(* Logix 5000 AddOnInstructionDefinition export Banner_TL50Select_Param_v4; software revision 33.00 *)

TYPE Banner_IOL_Port_v4 :   // UDT that has all of the data items necessary to communicate with a specific Port on a IO-Link Master
STRUCT
   Port_Controlled : INT;   // Each bit represents a port on an IO-Link Master. Set to 1 to tell AOI to control that port.
   Port_Activate : INT;   // Each bit represents a port on an IO-Link Master. When ON that port will process any commands in queue.
   Port_Read : INT;   // Each bit represents a port on an IO-Link Master. Used to determine when device AOI has requested a Read command.
   Port_Write : INT;   // Each bit represents a port on an IO-Link Master. Used to determine when device AOI has requested a Write command.
   Port_RW_Complete : INT;   // Each bit represents a port on an IO-Link Master. Tells device AOI that Read or Write request has been completed.
   Port_Device_Read : INT;
   Data_Transfer : SINT[190];   // Array to transfer data from IO-Master to device AOIs.
END_STRUCT
END_TYPE

TYPE Banner_TL50Select_Basic_SP_v4 :   // Basic parameters for a TL50 Pro Select segment.
STRUCT
   Basic_Color : SINT;   // 0 = Green, 1 = Red, 2 = Orange, 3 = Amber, 4 = Yellow, 5 = Lime Green, 6 = Spring Green, 7 = Cyan, 8 = Sky Blue, 9 = Blue, 10 = Violet, 11 = Magenta, 12 = Rose, 13 = White, 14 = Custom, 15 = Custom 2
   Basic_Speed : SINT;   // 0 = Medium, 1 = Fast, 2 = Slow, 3 = Custom
   Animation : SINT;   // 0 = Off, 1 = Steady, 2 = Flash, 3 = Two Color, 4 = Half/Half, 5 = Half/Half Rotate, 6 = Chase, 7 = Intesnity Sweep
   Animation_Color_1 : INT;   // 0 = Green, 1 = Red, 2 = Orange, 3 = Amber, 4 = Yellow, 5 = Lime Green, 6 = Spring Green, 7 = Cyan, 8 = Sky Blue, 9 = Blue, 10 = Violet, 11 = Magenta, 12 = Rose, 13 = White, 14 = Custom, 15 = Custom 2
   Animation_Color_1_Intensity : SINT;   // 0 = High, 1 = Low, 2 = Medium, 3 = Off, 4 = Custom
   Animation_Speed : SINT;   // 0 = Medium, 1 = Fasr, 2 = Slow, 3 = Custom
   Animation_Pattern : SINT;   // 0 = Normal, 1 = Strobe, 2 = Three Pulse, 3 = SOS, 4 = Random
   Animation_Color_2 : INT;   // 0 = Green, 1 = Red, 2 = Orange, 3 = Amber, 4 = Yellow, 5 = Lime Green, 6 = Spring Green, 7 = Cyan, 8 = Sky Blue, 9 = Blue, 10 = Violet, 11 = Magenta, 12 = Rose, 13 = White, 14 = Custom, 15 = Custom 2
   Animation_Color_2_Intensity : SINT;   // 0 = High, 1 = Low, 2 = Medium, 3 = Off, 4 = Custom
END_STRUCT
END_TYPE

TYPE Banner_TL50Select_RD_v4 :   // UDT that stores the Read Data for a TL50 Pro Select.
STRUCT
   Master_Cycle_Time : INT;
   Min_Cycle_Time : INT;
   M_Sequence_Capability : INT;
   IO_Link_Version_ID : INT;
   Process_Data_Input_Length : INT;
   Process_Data_Output_Length : INT;
   Combined_Vendor_ID : DINT;   // IO-Link Vendor ID
   Vendor_ID1 : INT;
   Vendor_ID2 : INT;
   Combined_Device_ID : DINT;   // IO-Link Device ID
   Device_ID1 : INT;
   Device_ID2 : INT;
   Device_ID3 : INT;
   Serial_Number : STRING;
END_STRUCT
END_TYPE

TYPE Banner_TL50Select_v4 :   // All of the parameters for a TL50 Pro Select.
STRUCT
   Initial_Global_Read : BOOL;   // Determines if all of the IO-Link data has been read into the PLC yet
   Command : INT;   // Value placed in here will activate a read or write to a specifc IO-Link Index
   Read : Banner_TL50Select_RD_v4;   // Read Only Data
   Write : Banner_TL50Select_WD_v4;   // Write Data
   Archive_Data : Banner_TL50Select_WD_v4;   // Archive of the Write Data
   Reset : BOOL;   // Resets AOI. This will force a complete parameter read of the sensor.
END_STRUCT
END_TYPE

TYPE Banner_TL50Select_WD_v4 :   // UDT that stores the Write Data for a TL50 Pro Select.
STRUCT
   System_Command : INT;   // See IODD file for list of commands that can be activated via the System Command interface
   Parameter_Access_Lock : SINT;   // Write access to all parameters is prohibited while value is 1. Only this parameter can be adjusted when value is 1.
   Data_Storage_Lock : SINT;   // Automatic data storage is disabled when this value is equal to 1. Read access is not affected.
   Local_Parameterization_Lock : SINT;   // Parameterization via local control elements on device is disabled.
   Local_User_Interface_Lock : SINT;   // Operation of local user interface is disabled.
   Operating_Mode_Selection : SINT;   // 0 = Basic Mode, 1 = Advanced Mode, 2= Run Mode, 3 = Level Mode
   Segment_Basic : Banner_TL50Select_Basic_SP_v4[5];
   Restrict_to_Gamut : SINT;   // 0 = Off, 1 = On
   Number_of_Segments_for_Scroll_and_Bounce : INT;   // 0 to 10
   Custom_Flash_Rate : INT;   // .5 to 20 Hz (range 5 to 200)
   Custom_Intensity : INT;   // 0 to 100%
   Custom_1_Red : INT;   // 0 to 255. Value of the Red portion of the RGB color value for Custom 1
   Custom_1_Green : INT;   // 0 to 255. Value of the Green portion of the RGB color value for Custom 1.
   Custom_1_Blue : INT;   // 0 to 255. Value of the Blue portion of the RGB color value for Custom 1.
   Custom_2_Red : INT;   // 0 to 255. Value of the Red portion of the RGB color value for Custom 2.
   Custom_2_Green : INT;   // 0 to 255. Value of the Green portion of the RGB color value for Custom 2.
   Custom_2_Blue : INT;   // 0 to 255. Value of the Blue portion of the RGB color value for Custom 2.
   LM_Full_Scale_Value : DINT;
   LM_Base_Color : INT;   // 0 = Green, 1 = Red, 2 = Orange, 3 = Amber, 4 = Yellow, 5 = Lime Green, 6 = Spring Green, 7 = Cyan, 8 = Sky Blue, 9 = Blue, 10 = Violet, 11 = Magenta, 12 = Rose, 13 = White, 14 = Custom, 15 = Custom 2
   LM_Base_Intensity : SINT;   // 0 = High, 1 = Low, 2 = Medium, 3 = Off, 4 = Custom
   LM_Base_State : SINT;   // 0 = Steady, 1 = Flashing
   LM_Threshold_Type : SINT;   // 0 = None, 1 = Low, 2 = High, 3 = High and Low
   LM_Low_Threshold_Value : DINT;
   LM_Low_Threshold_Color : INT;   // 0 = Green, 1 = Red, 2 = Orange, 3 = Amber, 4 = Yellow, 5 = Lime Green, 6 = Spring Green, 7 = Cyan, 8 = Sky Blue, 9 = Blue, 10 = Violet, 11 = Magenta, 12 = Rose, 13 = White, 14 = Custom, 15 = Custom 2
   LM_Low_Threshold_Intensity : SINT;   // 0 = High, 1 = Low, 2 = Medium, 3 = Off, 4 = Custom
   LM_Low_Threshold_State : SINT;   // 0 = Steady, 1 = Flashing
   LM_High_Threshold_Value : DINT;
   LM_High_Threshold_Color : INT;   // 0 = Green, 1 = Red, 2 = Orange, 3 = Amber, 4 = Yellow, 5 = Lime Green, 6 = Spring Green, 7 = Cyan, 8 = Sky Blue, 9 = Blue, 10 = Violet, 11 = Magenta, 12 = Rose, 13 = White, 14 = Custom, 15 = Custom 2
   LM_High_Threshold_Intensity : SINT;   // 0 = High, 1 = Low, 2 = Medium, 3 = Off, 4 = Custom
   LM_High_Threshold_State : SINT;   // 0 = Steady, 1 = Flashing
   LM_Flash_Rate : SINT;   // 0 = Medium, 1 = Fast, 2 = Slow, 3 = Custom
   LM_Dominance : SINT;   // 0 = Dominant, 1 = Non-Dominant
   LM_Subsegment_Style : SINT;   // 0 = Steady, 1 = Flashing, 2 = Analog
   LM_Background_Color : SINT;   // 0 = Green, 1 = Red, 2 = Orange, 3 = Amber, 4 = Yellow, 5 = Lime Green, 6 = Spring Green, 7 = Cyan, 8 = Sky Blue, 9 = Blue, 10 = Violet, 11 = Magenta, 12 = Rose, 13 = White, 14 = Custom, 15 = Custom 2
   LM_Background_Intensity : SINT;   // 0 = High, 1 = Low, 2 = Medium, 3 = Off, 4 = Custom
   LM_Orientation : SINT;   // 0 = Steady, 1 = Flashing
END_STRUCT
END_TYPE

ADD_ON_INSTRUCTION Banner_TL50Select_Param_v4   (* revision 4.1, vendor Banner Engineering *)
// AOI to read and write parameter data to an IO-Link TL50 Pro Select.
VAR_IN_OUT
   TL50_Pro : Banner_TL50Select_v4; {required}
   Port_Data : Banner_IOL_Port_v4; {required}
END_VAR
VAR_INPUT
   Port : INT; {required}   // Port Number that device is plugged into.
END_VAR
VAR
   Local_Control : DINT; {access None}
   Global_Read_Command_Value : INT; {access None}
   Global_Write_Command_Value : INT; {access None}
   Command_Being_Processed : BOOL; {access None}
   Update_Archive : BOOL; {access None}
   Index_Write_Inprocess : DINT; {access None}
   Index_Write_Control : DINT; {access None}
   Inprocess_Index : DINT; {access None}
   Index_R_Segment : DINT; {access None}
   BS_Index : DINT; {access None}
   Index_W_Segment : DINT; {access None}
   SB_W_Index : DINT; {access None}
   Index_Segment_Read : DINT; {access None}
END_VAR

ROUTINE Logic   (* ladder *)
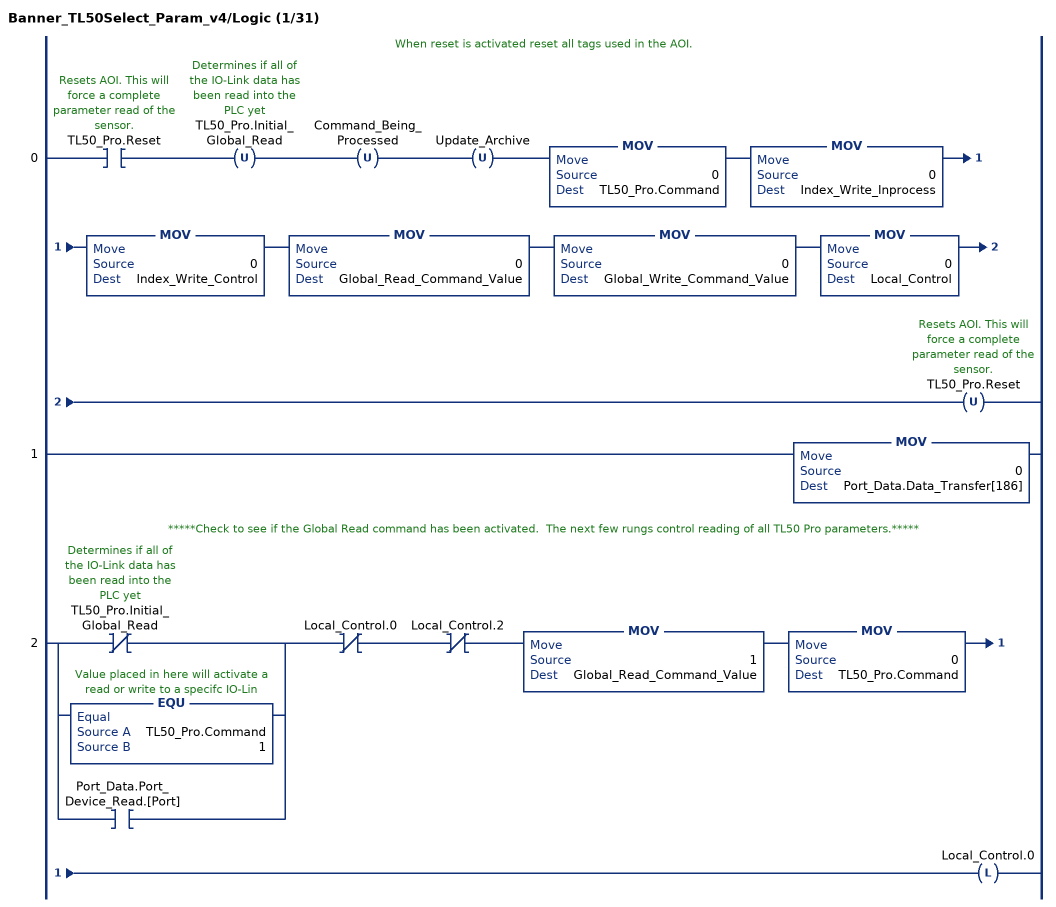
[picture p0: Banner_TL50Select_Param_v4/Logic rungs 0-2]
   // When reset is activated reset all tags used in the AOI.
   0: XIC(TL50_Pro.Reset)OTU(TL50_Pro.Initial_Global_Read)OTU(Command_Being_Processed)OTU(Update_Archive)MOV(0,TL50_Pro.Command)MOV(0,Index_Write_Inprocess)MOV(0,Index_Write_Control)MOV(0,Global_Read_Command_Value)MOV(0,Global_Write_Command_Value)MOV(0,Local_Control)OTU(TL50_Pro.Reset);
   1: MOV(0,Port_Data.Data_Transfer[186]);
   // *****Check to see if the Global Read command has been activated.  The next few rungs control reading of all TL50 Pro parameters.*****
   2: [XIO(TL50_Pro.Initial_Global_Read) ,EQU(TL50_Pro.Command,1) ,XIC(Port_Data.Port_Device_Read.[Port]) ]XIO(Local_Control.0)XIO(Local_Control.2)MOV(1,Global_Read_Command_Value)MOV(0,TL50_Pro.Command)OTL(Local_Control.0);
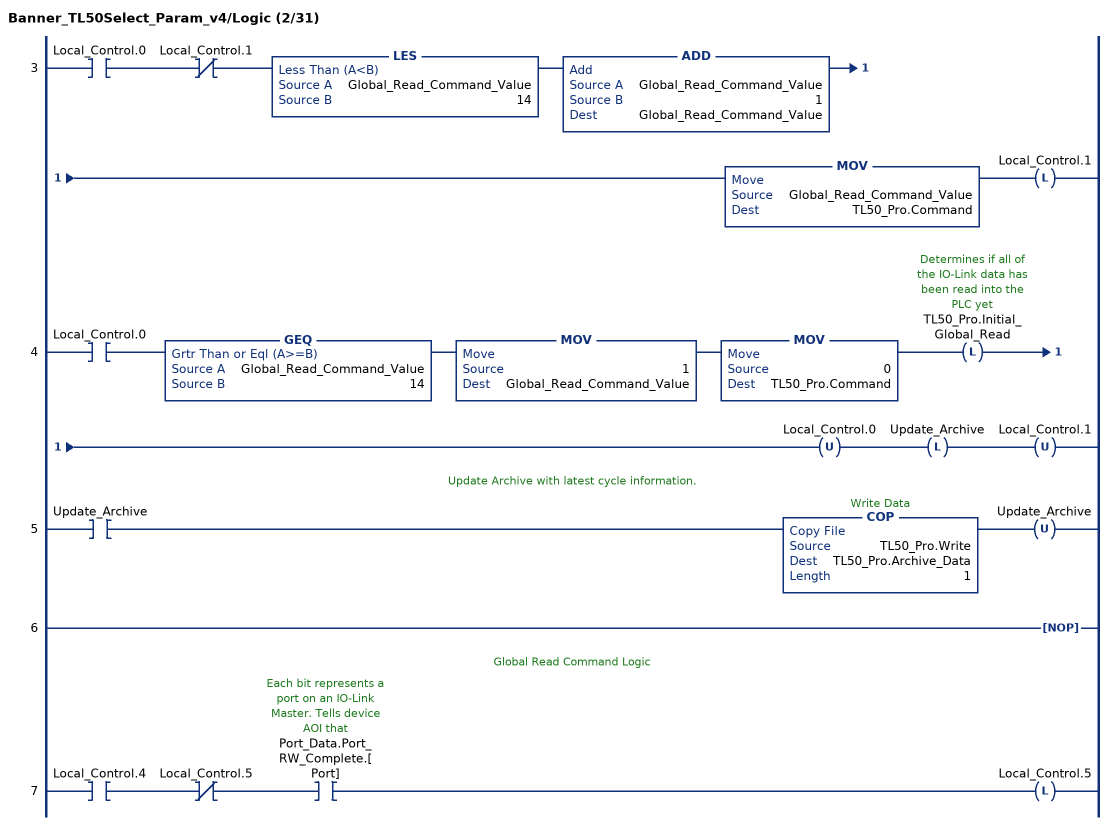
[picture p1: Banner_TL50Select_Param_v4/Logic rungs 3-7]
   3: XIC(Local_Control.0)XIO(Local_Control.1)LES(Global_Read_Command_Value,14)ADD(Global_Read_Command_Value,1,Global_Read_Command_Value)MOV(Global_Read_Command_Value,TL50_Pro.Command)OTL(Local_Control.1);
   4: XIC(Local_Control.0)GEQ(Global_Read_Command_Value,14)MOV(1,Global_Read_Command_Value)MOV(0,TL50_Pro.Command)OTL(TL50_Pro.Initial_Global_Read)OTU(Local_Control.0)OTL(Update_Archive)OTU(Local_Control.1);
   // Update Archive with latest cycle information.
   5: XIC(Update_Archive)COP(TL50_Pro.Write,TL50_Pro.Archive_Data,1)OTU(Update_Archive);
   6: NOP();
   // Global Read Command Logic
   7: XIC(Local_Control.4)XIO(Local_Control.5)XIC(Port_Data.Port_RW_Complete.[Port])OTL(Local_Control.5);
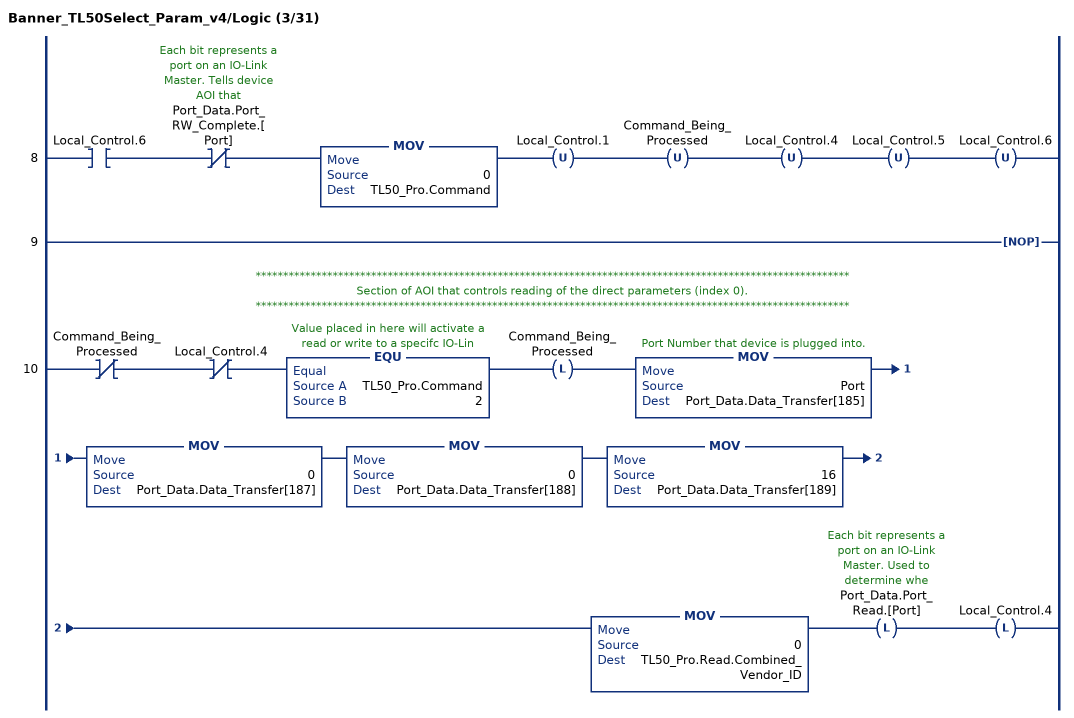
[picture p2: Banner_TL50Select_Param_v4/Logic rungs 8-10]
   8: XIC(Local_Control.6)XIO(Port_Data.Port_RW_Complete.[Port])MOV(0,TL50_Pro.Command)OTU(Local_Control.1)OTU(Command_Being_Processed)OTU(Local_Control.4)OTU(Local_Control.5)OTU(Local_Control.6);
   9: NOP();
   // ************************************************************************************************************
   // Section of AOI that controls reading of the direct parameters (index 0).
   // ************************************************************************************************************
   10: XIO(Command_Being_Processed)XIO(Local_Control.4)EQU(TL50_Pro.Command,2)OTL(Command_Being_Processed)MOV(Port,Port_Data.Data_Transfer[185])MOV(0,Port_Data.Data_Transfer[187])MOV(0,Port_Data.Data_Transfer[188])MOV(16,Port_Data.Data_Transfer[189])MOV(0,TL50_Pro.Read.Combined_Vendor_ID)OTL(Port_Data.Port_Read.[Port])OTL(Local_Control.4);
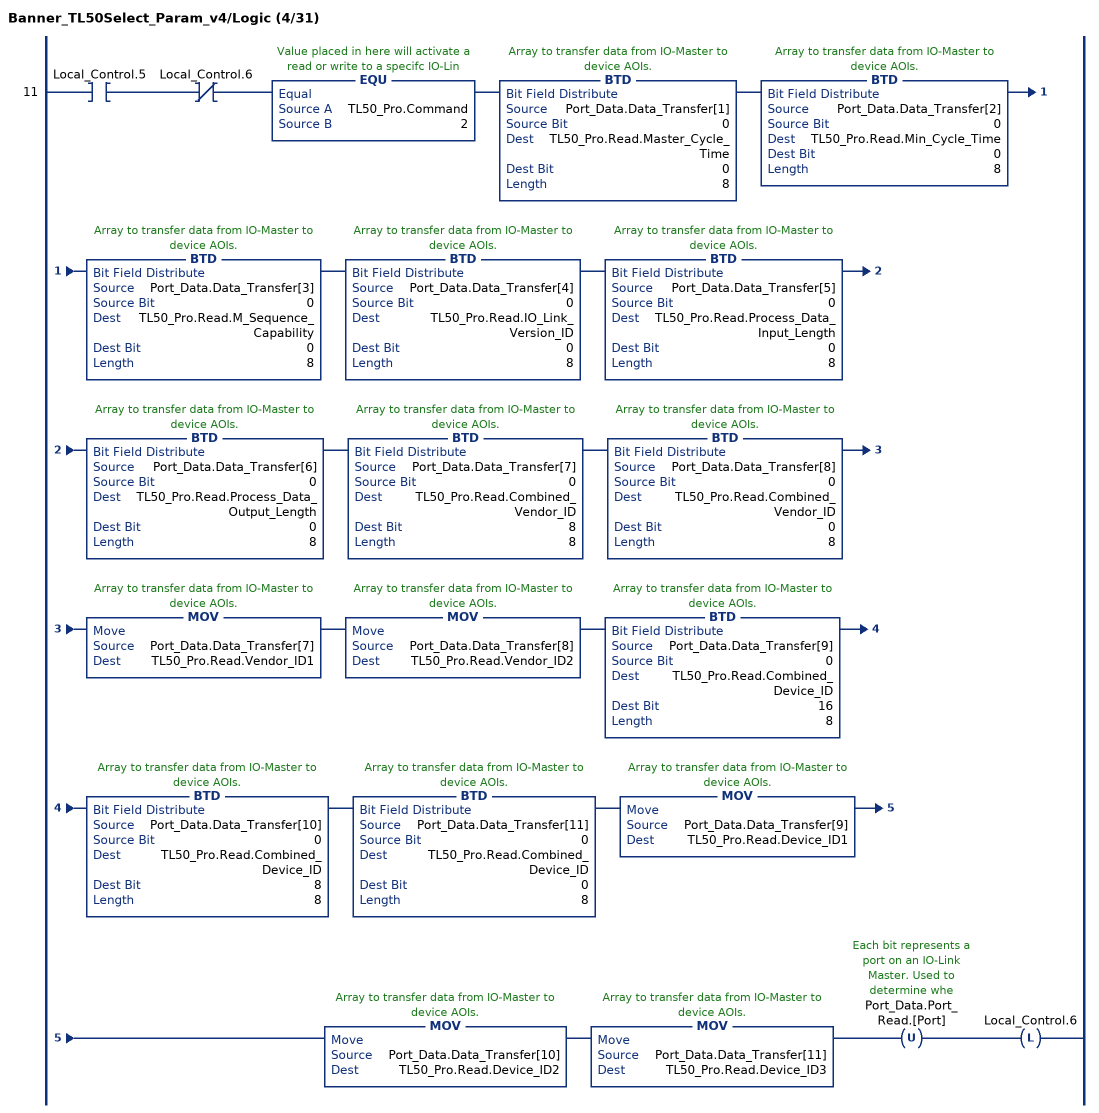
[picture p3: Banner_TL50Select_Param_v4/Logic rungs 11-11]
   11: XIC(Local_Control.5)XIO(Local_Control.6)EQU(TL50_Pro.Command,2)BTD(Port_Data.Data_Transfer[1],0,TL50_Pro.Read.Master_Cycle_Time,0,8)BTD(Port_Data.Data_Transfer[2],0,TL50_Pro.Read.Min_Cycle_Time,0,8)BTD(Port_Data.Data_Transfer[3],0,TL50_Pro.Read.M_Sequence_Capability,0,8)BTD(Port_Data.Data_Transfer[4],0,TL50_Pro.Read.IO_Link_Version_ID,0,8)BTD(Port_Data.Data_Transfer[5],0,TL50_Pro.Read.Process_Data_Input_Length,0,8)BTD(Port_Data.Data_Transfer[6],0,TL50_Pro.Read.Process_Data_Output_Length,0,8)BTD(Port_Data.Data_Transfer[7],0,TL50_Pro.Read.Combined_Vendor_ID,8,8)BTD(Port_Data.Data_Transfer[8],0,TL50_Pro.Read.Combined_Vendor_ID,0,8)MOV(Port_Data.Data_Transfer[7],TL50_Pro.Read.Vendor_ID1)MOV(Port_Data.Data_Transfer[8],TL50_Pro.Read.Vendor_ID2)BTD(Port_Data.Data_Transfer[9],0,TL50_Pro.Read.Combined_Device_ID,16,8)BTD(Port_Data.Data_Transfer[10],0,TL50_Pro.Read.Combined_Device_ID,8,8)BTD(Port_Data.Data_Transfer[11],0,TL50_Pro.Read.Combined_Device_ID,0,8)MOV(Port_Data.Data_Transfer[9],TL50_Pro.Read.Device_ID1)MOV(Port_Data.Data_Transfer[10],TL50_Pro.Read.Device_ID2)MOV(Port_Data.Data_Transfer[11],TL50_Pro.Read.Device_ID3)OTU(Port_Data.Port_Read.[Port])OTL(Local_Control.6);
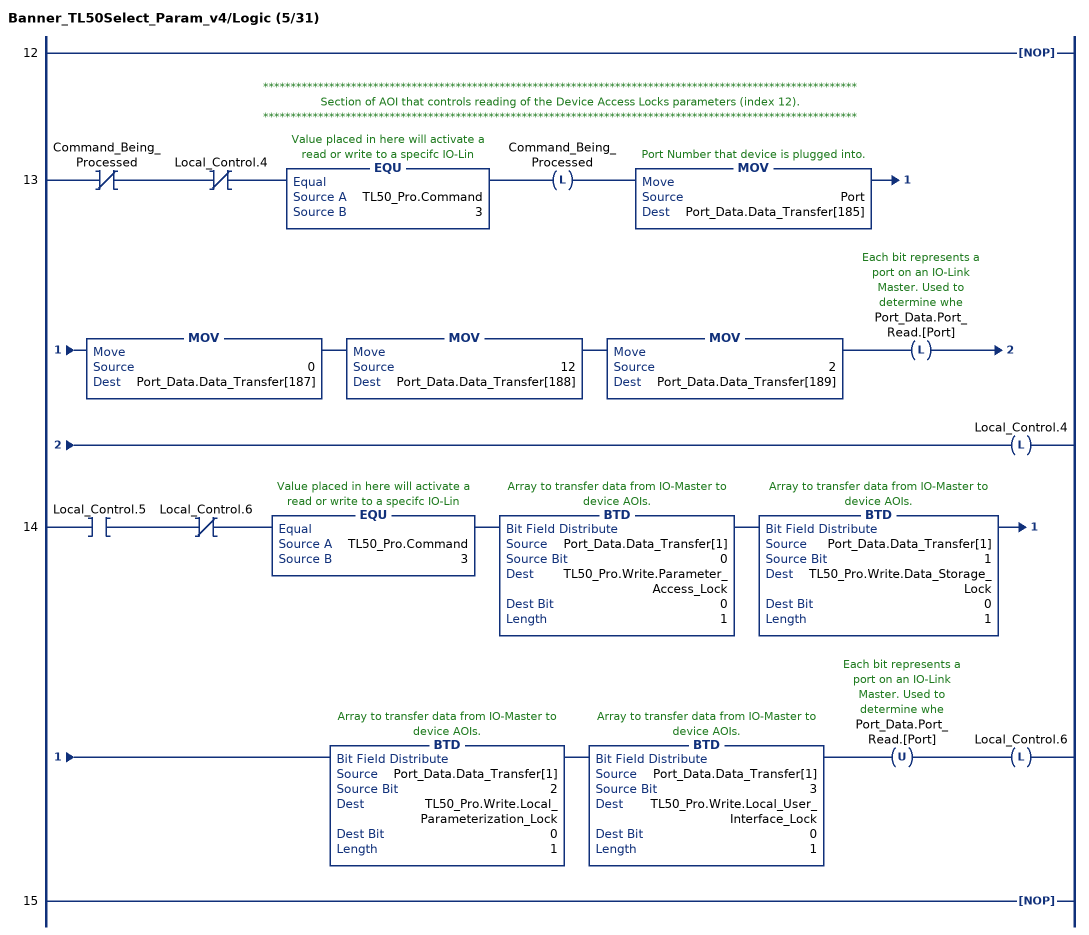
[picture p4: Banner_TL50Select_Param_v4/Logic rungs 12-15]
   12: NOP();
   // ************************************************************************************************************
   // Section of AOI that controls reading of the Device Access Locks parameters (index 12).
   // ************************************************************************************************************
   13: XIO(Command_Being_Processed)XIO(Local_Control.4)EQU(TL50_Pro.Command,3)OTL(Command_Being_Processed)MOV(Port,Port_Data.Data_Transfer[185])MOV(0,Port_Data.Data_Transfer[187])MOV(12,Port_Data.Data_Transfer[188])MOV(2,Port_Data.Data_Transfer[189])OTL(Port_Data.Port_Read.[Port])OTL(Local_Control.4);
   14: XIC(Local_Control.5)XIO(Local_Control.6)EQU(TL50_Pro.Command,3)BTD(Port_Data.Data_Transfer[1],0,TL50_Pro.Write.Parameter_Access_Lock,0,1)BTD(Port_Data.Data_Transfer[1],1,TL50_Pro.Write.Data_Storage_Lock,0,1)BTD(Port_Data.Data_Transfer[1],2,TL50_Pro.Write.Local_Parameterization_Lock,0,1)BTD(Port_Data.Data_Transfer[1],3,TL50_Pro.Write.Local_User_Interface_Lock,0,1)OTU(Port_Data.Port_Read.[Port])OTL(Local_Control.6);
   15: NOP();
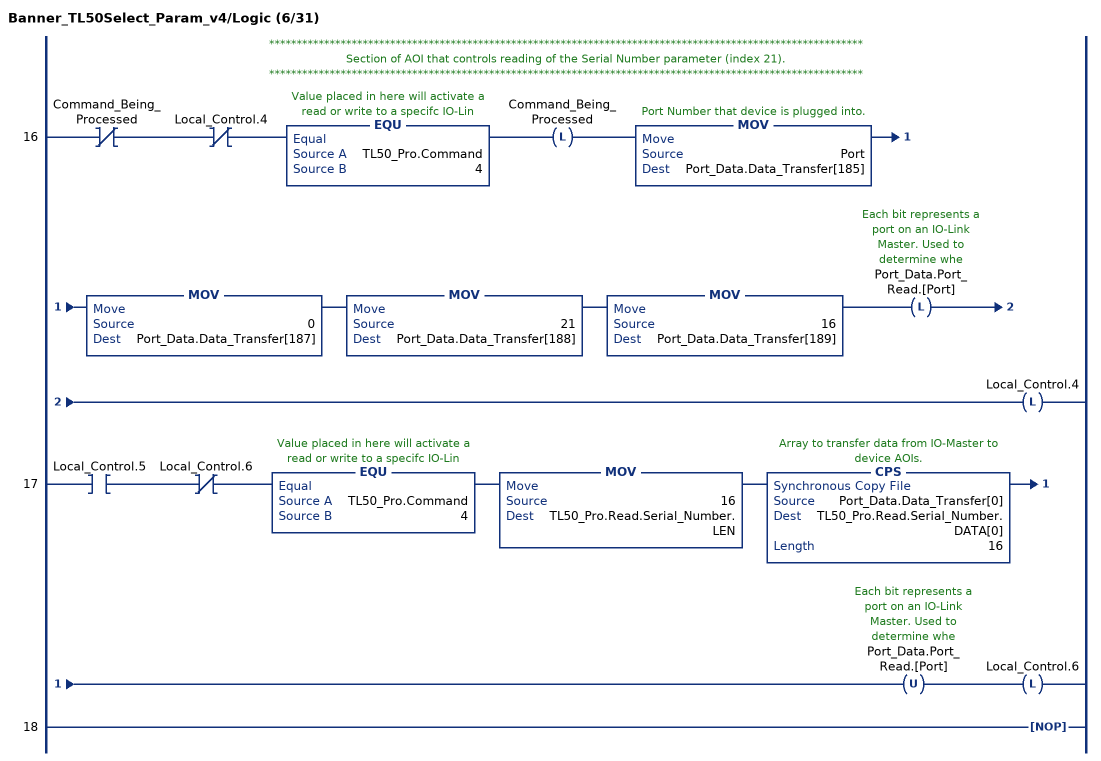
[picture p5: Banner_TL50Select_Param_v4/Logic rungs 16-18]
   // ************************************************************************************************************
   // Section of AOI that controls reading of the Serial Number parameter (index 21).
   // ************************************************************************************************************
   16: XIO(Command_Being_Processed)XIO(Local_Control.4)EQU(TL50_Pro.Command,4)OTL(Command_Being_Processed)MOV(Port,Port_Data.Data_Transfer[185])MOV(0,Port_Data.Data_Transfer[187])MOV(21,Port_Data.Data_Transfer[188])MOV(16,Port_Data.Data_Transfer[189])OTL(Port_Data.Port_Read.[Port])OTL(Local_Control.4);
   17: XIC(Local_Control.5)XIO(Local_Control.6)EQU(TL50_Pro.Command,4)MOV(16,TL50_Pro.Read.Serial_Number.LEN)CPS(Port_Data.Data_Transfer[0],TL50_Pro.Read.Serial_Number.DATA[0],16)OTU(Port_Data.Port_Read.[Port])OTL(Local_Control.6);
   18: NOP();
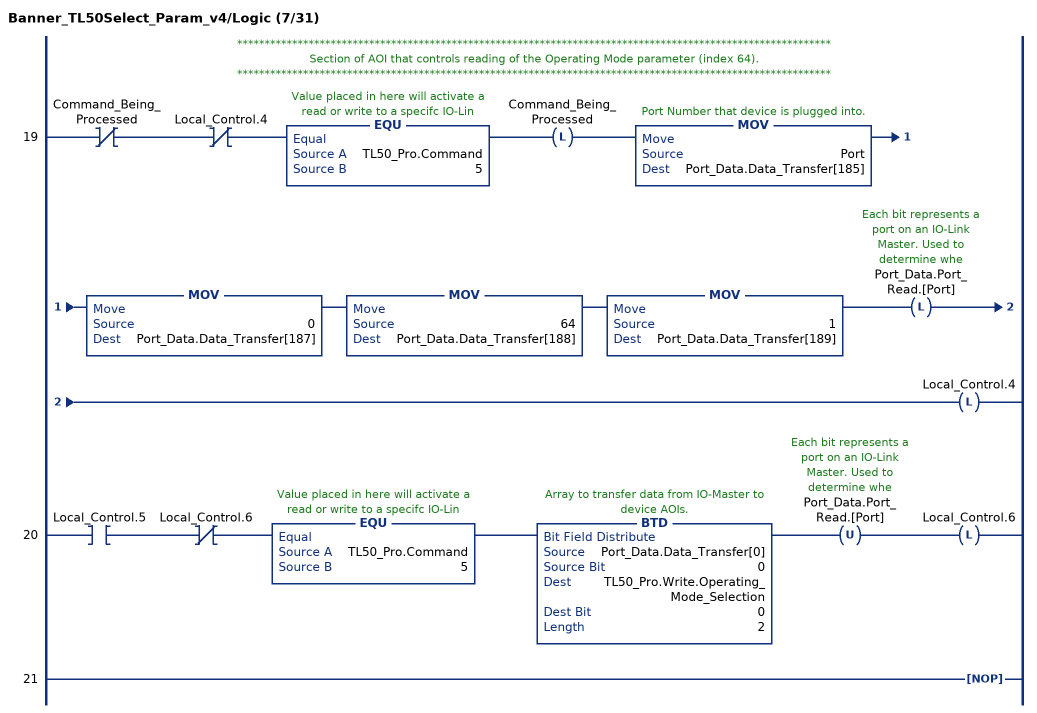
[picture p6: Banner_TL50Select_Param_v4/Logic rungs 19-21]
   // ************************************************************************************************************
   // Section of AOI that controls reading of the Operating Mode parameter (index 64).
   // ************************************************************************************************************
   19: XIO(Command_Being_Processed)XIO(Local_Control.4)EQU(TL50_Pro.Command,5)OTL(Command_Being_Processed)MOV(Port,Port_Data.Data_Transfer[185])MOV(0,Port_Data.Data_Transfer[187])MOV(64,Port_Data.Data_Transfer[188])MOV(1,Port_Data.Data_Transfer[189])OTL(Port_Data.Port_Read.[Port])OTL(Local_Control.4);
   20: XIC(Local_Control.5)XIO(Local_Control.6)EQU(TL50_Pro.Command,5)BTD(Port_Data.Data_Transfer[0],0,TL50_Pro.Write.Operating_Mode_Selection,0,2)OTU(Port_Data.Port_Read.[Port])OTL(Local_Control.6);
   21: NOP();
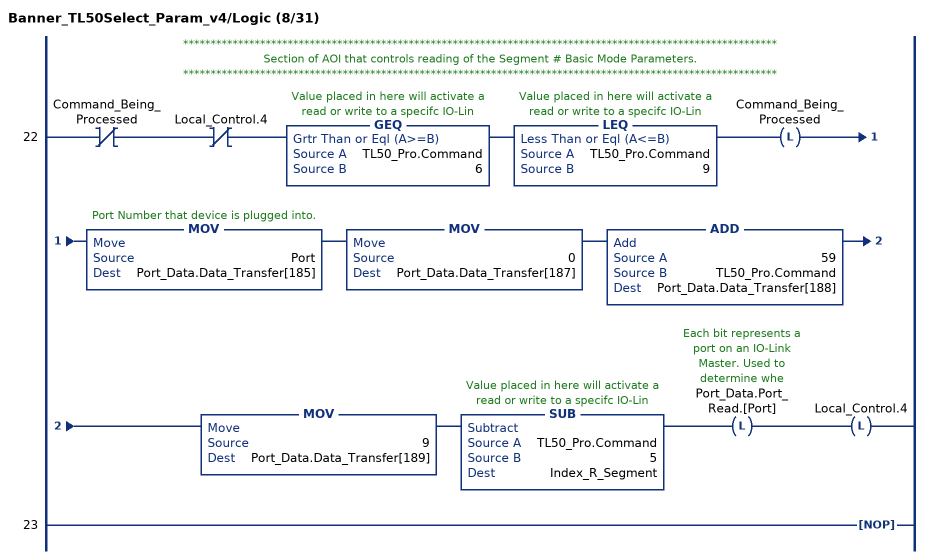
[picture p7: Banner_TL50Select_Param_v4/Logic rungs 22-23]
   // ************************************************************************************************************
   // Section of AOI that controls reading of the Segment # Basic Mode Parameters.
   // ************************************************************************************************************
   22: XIO(Command_Being_Processed)XIO(Local_Control.4)GEQ(TL50_Pro.Command,6)LEQ(TL50_Pro.Command,9)OTL(Command_Being_Processed)MOV(Port,Port_Data.Data_Transfer[185])MOV(0,Port_Data.Data_Transfer[187])ADD(59,TL50_Pro.Command,Port_Data.Data_Transfer[188])MOV(9,Port_Data.Data_Transfer[189])SUB(TL50_Pro.Command,5,Index_R_Segment)OTL(Port_Data.Port_Read.[Port])OTL(Local_Control.4);
   23: NOP();
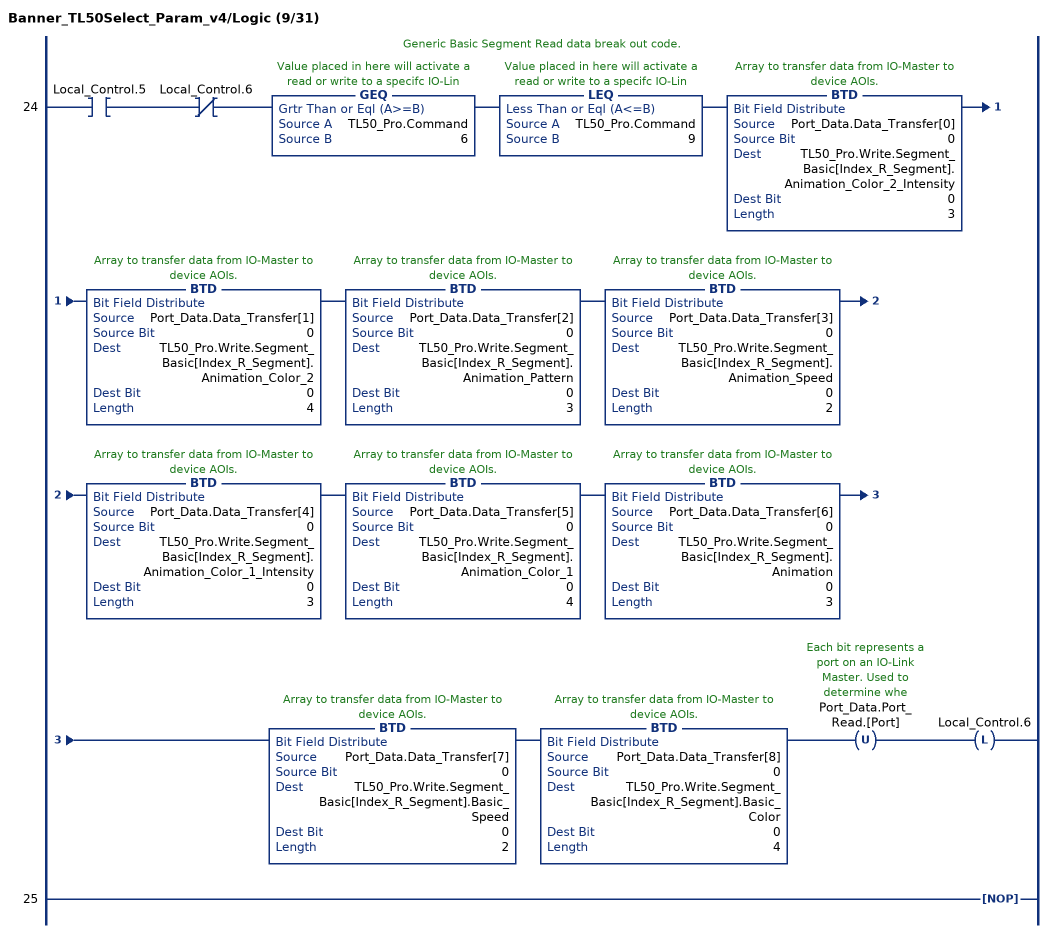
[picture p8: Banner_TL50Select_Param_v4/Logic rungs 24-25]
   // Generic Basic Segment Read data break out code.
   24: XIC(Local_Control.5)XIO(Local_Control.6)GEQ(TL50_Pro.Command,6)LEQ(TL50_Pro.Command,9)BTD(Port_Data.Data_Transfer[0],0,TL50_Pro.Write.Segment_Basic[Index_R_Segment].Animation_Color_2_Intensity,0,3)BTD(Port_Data.Data_Transfer[1],0,TL50_Pro.Write.Segment_Basic[Index_R_Segment].Animation_Color_2,0,4)BTD(Port_Data.Data_Transfer[2],0,TL50_Pro.Write.Segment_Basic[Index_R_Segment].Animation_Pattern,0,3)BTD(Port_Data.Data_Transfer[3],0,TL50_Pro.Write.Segment_Basic[Index_R_Segment].Animation_Speed,0,2)BTD(Port_Data.Data_Transfer[4],0,TL50_Pro.Write.Segment_Basic[Index_R_Segment].Animation_Color_1_Intensity,0,3)BTD(Port_Data.Data_Transfer[5],0,TL50_Pro.Write.Segment_Basic[Index_R_Segment].Animation_Color_1,0,4)BTD(Port_Data.Data_Transfer[6],0,TL50_Pro.Write.Segment_Basic[Index_R_Segment].Animation,0,3)BTD(Port_Data.Data_Transfer[7],0,TL50_Pro.Write.Segment_Basic[Index_R_Segment].Basic_Speed,0,2)BTD(Port_Data.Data_Transfer[8],0,TL50_Pro.Write.Segment_Basic[Index_R_Segment].Basic_Color,0,4)OTU(Port_Data.Port_Read.[Port])OTL(Local_Control.6);
   25: NOP();
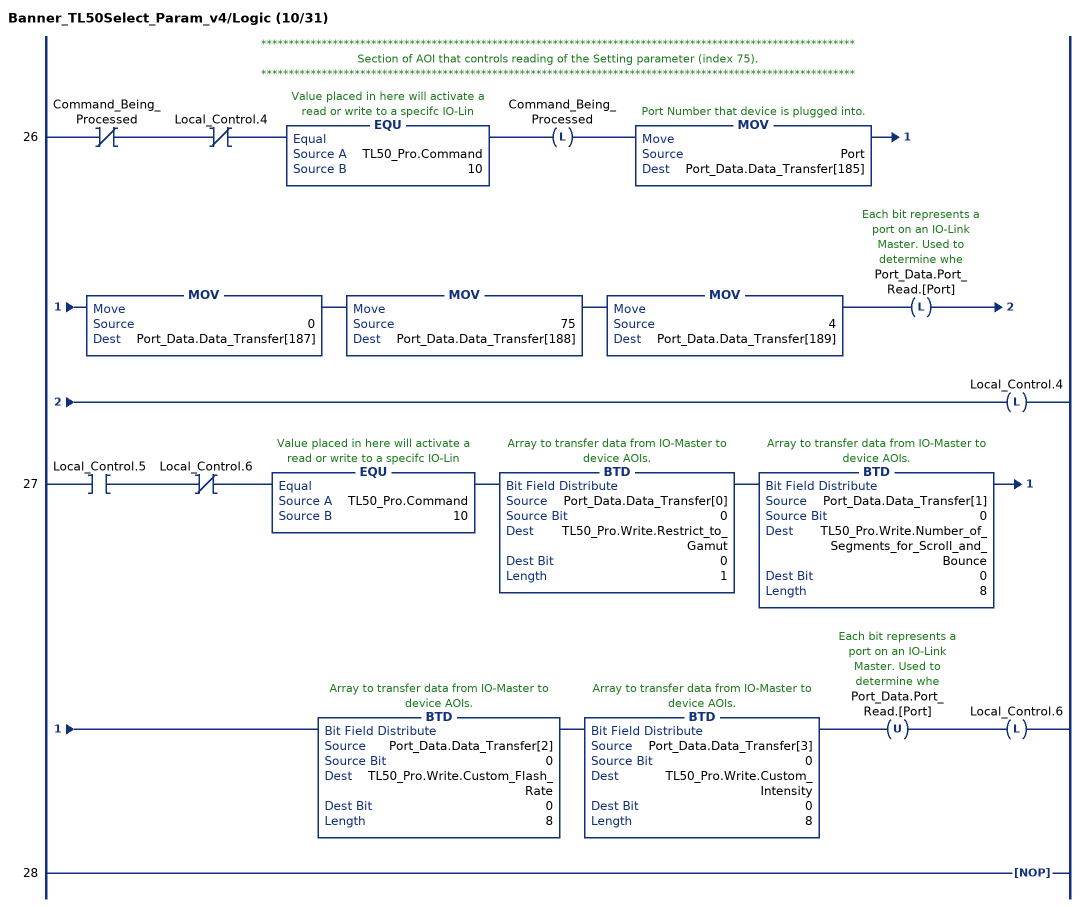
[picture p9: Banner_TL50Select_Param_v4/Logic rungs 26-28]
   // ************************************************************************************************************
   // Section of AOI that controls reading of the Setting parameter (index 75).
   // ************************************************************************************************************
   26: XIO(Command_Being_Processed)XIO(Local_Control.4)EQU(TL50_Pro.Command,10)OTL(Command_Being_Processed)MOV(Port,Port_Data.Data_Transfer[185])MOV(0,Port_Data.Data_Transfer[187])MOV(75,Port_Data.Data_Transfer[188])MOV(4,Port_Data.Data_Transfer[189])OTL(Port_Data.Port_Read.[Port])OTL(Local_Control.4);
   27: XIC(Local_Control.5)XIO(Local_Control.6)EQU(TL50_Pro.Command,10)BTD(Port_Data.Data_Transfer[0],0,TL50_Pro.Write.Restrict_to_Gamut,0,1)BTD(Port_Data.Data_Transfer[1],0,TL50_Pro.Write.Number_of_Segments_for_Scroll_and_Bounce,0,8)BTD(Port_Data.Data_Transfer[2],0,TL50_Pro.Write.Custom_Flash_Rate,0,8)BTD(Port_Data.Data_Transfer[3],0,TL50_Pro.Write.Custom_Intensity,0,8)OTU(Port_Data.Port_Read.[Port])OTL(Local_Control.6);
   28: NOP();
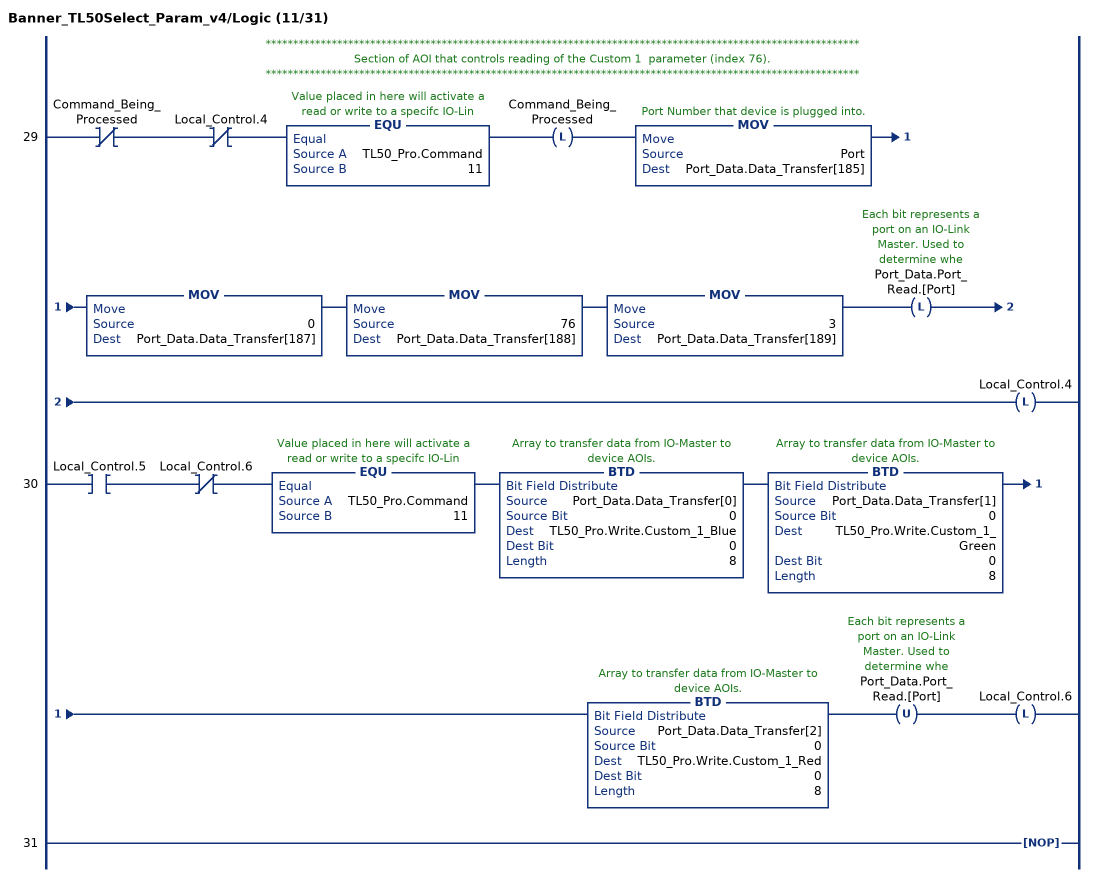
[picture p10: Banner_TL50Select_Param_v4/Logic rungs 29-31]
   // ************************************************************************************************************
   // Section of AOI that controls reading of the Custom 1  parameter (index 76).
   // ************************************************************************************************************
   29: XIO(Command_Being_Processed)XIO(Local_Control.4)EQU(TL50_Pro.Command,11)OTL(Command_Being_Processed)MOV(Port,Port_Data.Data_Transfer[185])MOV(0,Port_Data.Data_Transfer[187])MOV(76,Port_Data.Data_Transfer[188])MOV(3,Port_Data.Data_Transfer[189])OTL(Port_Data.Port_Read.[Port])OTL(Local_Control.4);
   30: XIC(Local_Control.5)XIO(Local_Control.6)EQU(TL50_Pro.Command,11)BTD(Port_Data.Data_Transfer[0],0,TL50_Pro.Write.Custom_1_Blue,0,8)BTD(Port_Data.Data_Transfer[1],0,TL50_Pro.Write.Custom_1_Green,0,8)BTD(Port_Data.Data_Transfer[2],0,TL50_Pro.Write.Custom_1_Red,0,8)OTU(Port_Data.Port_Read.[Port])OTL(Local_Control.6);
   31: NOP();
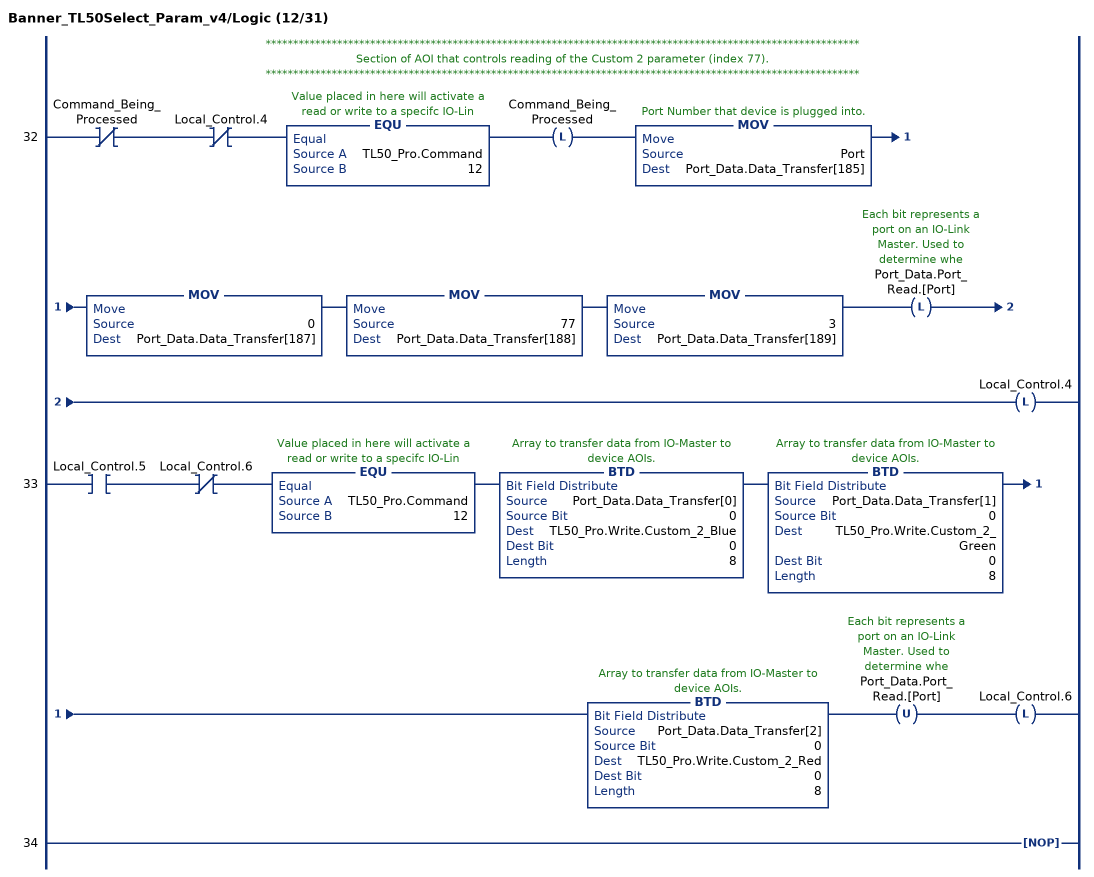
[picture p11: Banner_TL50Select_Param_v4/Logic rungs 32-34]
   // ************************************************************************************************************
   // Section of AOI that controls reading of the Custom 2 parameter (index 77).
   // ************************************************************************************************************
   32: XIO(Command_Being_Processed)XIO(Local_Control.4)EQU(TL50_Pro.Command,12)OTL(Command_Being_Processed)MOV(Port,Port_Data.Data_Transfer[185])MOV(0,Port_Data.Data_Transfer[187])MOV(77,Port_Data.Data_Transfer[188])MOV(3,Port_Data.Data_Transfer[189])OTL(Port_Data.Port_Read.[Port])OTL(Local_Control.4);
   33: XIC(Local_Control.5)XIO(Local_Control.6)EQU(TL50_Pro.Command,12)BTD(Port_Data.Data_Transfer[0],0,TL50_Pro.Write.Custom_2_Blue,0,8)BTD(Port_Data.Data_Transfer[1],0,TL50_Pro.Write.Custom_2_Green,0,8)BTD(Port_Data.Data_Transfer[2],0,TL50_Pro.Write.Custom_2_Red,0,8)OTU(Port_Data.Port_Read.[Port])OTL(Local_Control.6);
   34: NOP();
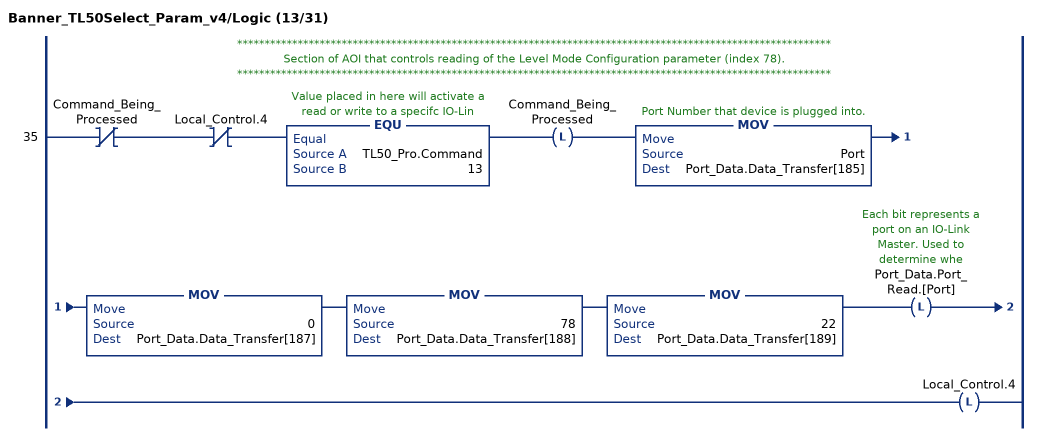
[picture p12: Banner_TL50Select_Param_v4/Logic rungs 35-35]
   // ************************************************************************************************************
   // Section of AOI that controls reading of the Level Mode Configuration parameter (index 78).
   // ************************************************************************************************************
   35: XIO(Command_Being_Processed)XIO(Local_Control.4)EQU(TL50_Pro.Command,13)OTL(Command_Being_Processed)MOV(Port,Port_Data.Data_Transfer[185])MOV(0,Port_Data.Data_Transfer[187])MOV(78,Port_Data.Data_Transfer[188])MOV(22,Port_Data.Data_Transfer[189])OTL(Port_Data.Port_Read.[Port])OTL(Local_Control.4);
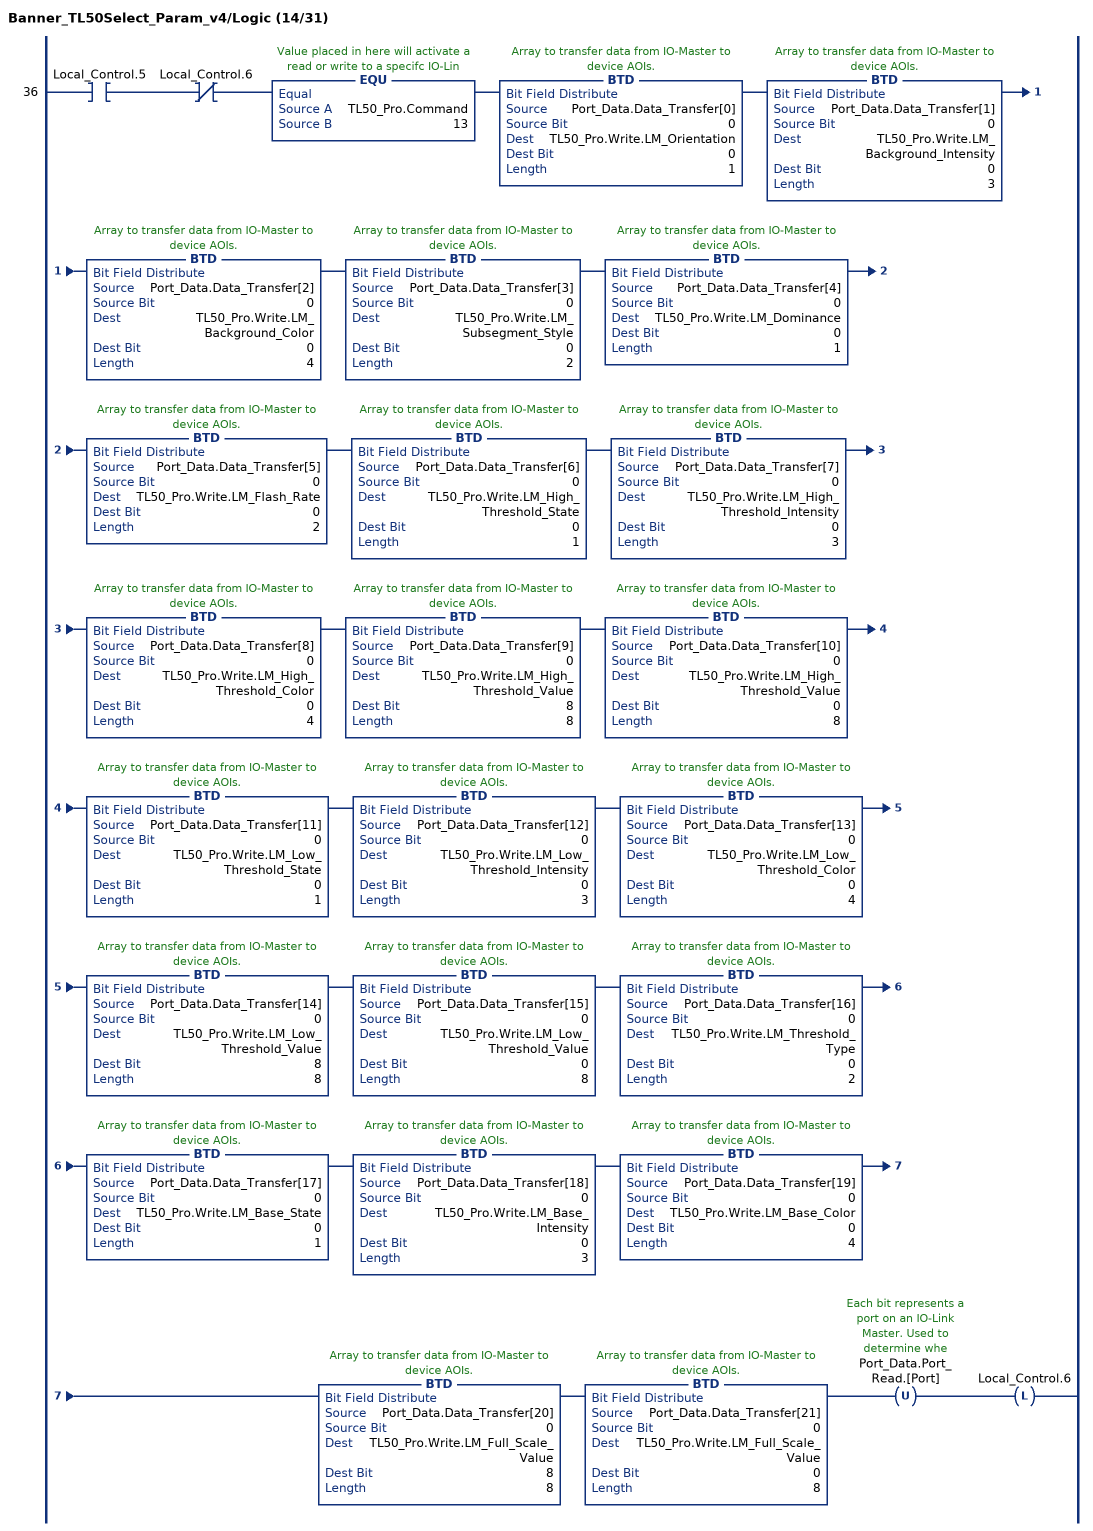
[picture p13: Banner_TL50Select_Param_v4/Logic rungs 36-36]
   36: XIC(Local_Control.5)XIO(Local_Control.6)EQU(TL50_Pro.Command,13)BTD(Port_Data.Data_Transfer[0],0,TL50_Pro.Write.LM_Orientation,0,1)BTD(Port_Data.Data_Transfer[1],0,TL50_Pro.Write.LM_Background_Intensity,0,3)BTD(Port_Data.Data_Transfer[2],0,TL50_Pro.Write.LM_Background_Color,0,4)BTD(Port_Data.Data_Transfer[3],0,TL50_Pro.Write.LM_Subsegment_Style,0,2)BTD(Port_Data.Data_Transfer[4],0,TL50_Pro.Write.LM_Dominance,0,1)BTD(Port_Data.Data_Transfer[5],0,TL50_Pro.Write.LM_Flash_Rate,0,2)BTD(Port_Data.Data_Transfer[6],0,TL50_Pro.Write.LM_High_Threshold_State,0,1)BTD(Port_Data.Data_Transfer[7],0,TL50_Pro.Write.LM_High_Threshold_Intensity,0,3)BTD(Port_Data.Data_Transfer[8],0,TL50_Pro.Write.LM_High_Threshold_Color,0,4)BTD(Port_Data.Data_Transfer[9],0,TL50_Pro.Write.LM_High_Threshold_Value,8,8)BTD(Port_Data.Data_Transfer[10],0,TL50_Pro.Write.LM_High_Threshold_Value,0,8)BTD(Port_Data.Data_Transfer[11],0,TL50_Pro.Write.LM_Low_Threshold_State,0,1)BTD(Port_Data.Data_Transfer[12],0,TL50_Pro.Write.LM_Low_Threshold_Intensity,0,3)BTD(Port_Data.Data_Transfer[13],0,TL50_Pro.Write.LM_Low_Threshold_Color,0,4)BTD(Port_Data.Data_Transfer[14],0,TL50_Pro.Write.LM_Low_Threshold_Value,8,8)BTD(Port_Data.Data_Transfer[15],0,TL50_Pro.Write.LM_Low_Threshold_Value,0,8)BTD(Port_Data.Data_Transfer[16],0,TL50_Pro.Write.LM_Threshold_Type,0,2)BTD(Port_Data.Data_Transfer[17],0,TL50_Pro.Write.LM_Base_State,0,1)BTD(Port_Data.Data_Transfer[18],0,TL50_Pro.Write.LM_Base_Intensity,0,3)BTD(Port_Data.Data_Transfer[19],0,TL50_Pro.Write.LM_Base_Color,0,4)BTD(Port_Data.Data_Transfer[20],0,TL50_Pro.Write.LM_Full_Scale_Value,8,8)BTD(Port_Data.Data_Transfer[21],0,TL50_Pro.Write.LM_Full_Scale_Value,0,8)OTU(Port_Data.Port_Read.[Port])OTL(Local_Control.6);
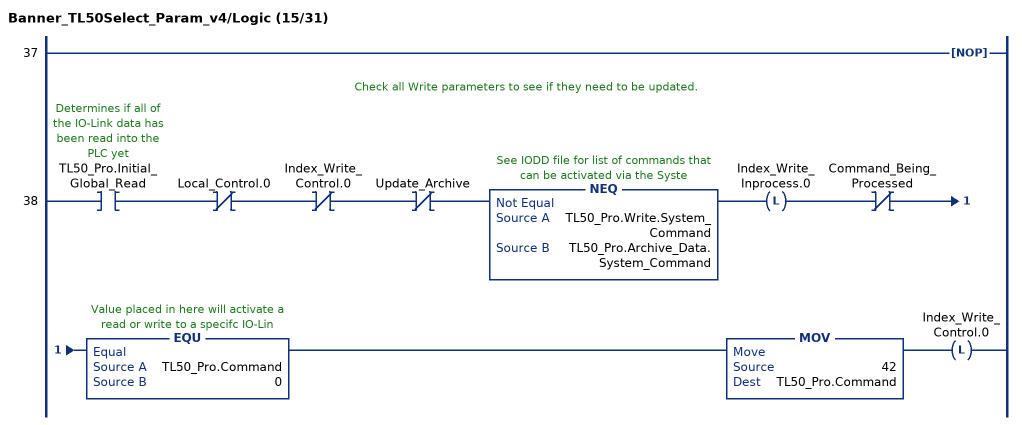
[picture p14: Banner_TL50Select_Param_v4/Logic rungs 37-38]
   37: NOP();
   // Check all Write parameters to see if they need to be updated.
   38: XIC(TL50_Pro.Initial_Global_Read)XIO(Local_Control.0)XIO(Index_Write_Control.0)XIO(Update_Archive)NEQ(TL50_Pro.Write.System_Command,TL50_Pro.Archive_Data.System_Command)OTL(Index_Write_Inprocess.0)XIO(Command_Being_Processed)EQU(TL50_Pro.Command,0)MOV(42,TL50_Pro.Command)OTL(Index_Write_Control.0);
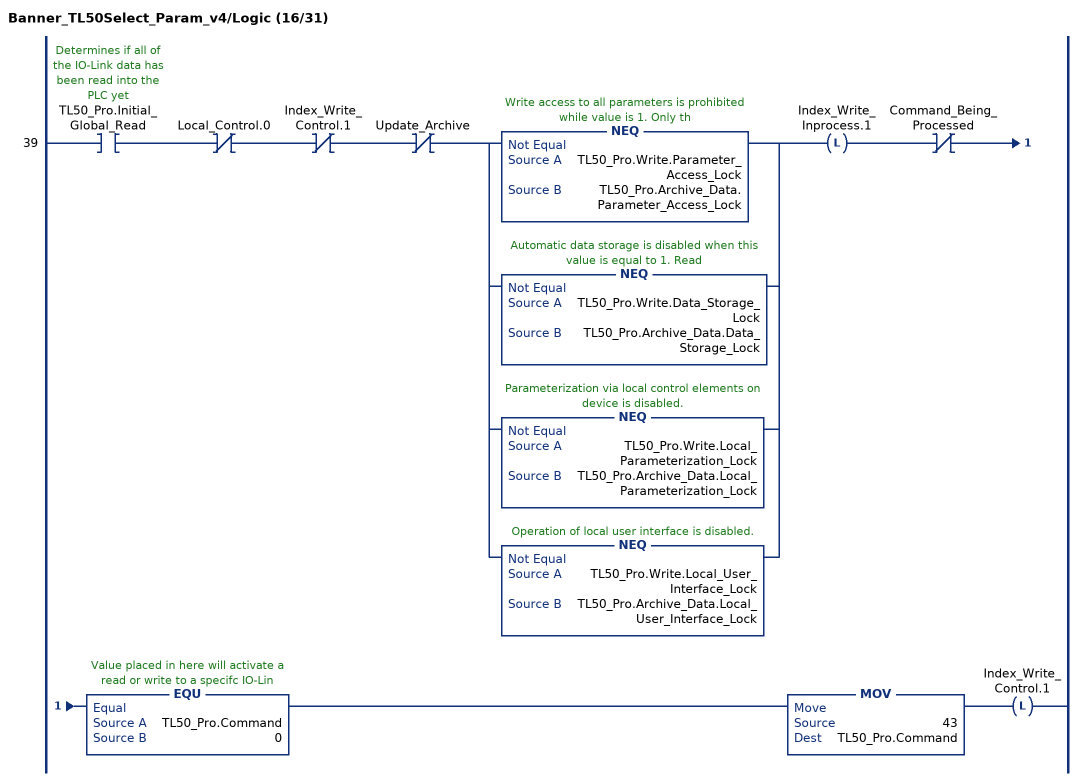
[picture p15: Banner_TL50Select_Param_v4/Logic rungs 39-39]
   39: XIC(TL50_Pro.Initial_Global_Read)XIO(Local_Control.0)XIO(Index_Write_Control.1)XIO(Update_Archive)[NEQ(TL50_Pro.Write.Parameter_Access_Lock,TL50_Pro.Archive_Data.Parameter_Access_Lock) ,NEQ(TL50_Pro.Write.Data_Storage_Lock,TL50_Pro.Archive_Data.Data_Storage_Lock) ,NEQ(TL50_Pro.Write.Local_Parameterization_Lock,TL50_Pro.Archive_Data.Local_Parameterization_Lock) ,NEQ(TL50_Pro.Write.Local_User_Interface_Lock,TL50_Pro.Archive_Data.Local_User_Interface_Lock) ]OTL(Index_Write_Inprocess.1)XIO(Command_Being_Processed)EQU(TL50_Pro.Command,0)MOV(43,TL50_Pro.Command)OTL(Index_Write_Control.1);
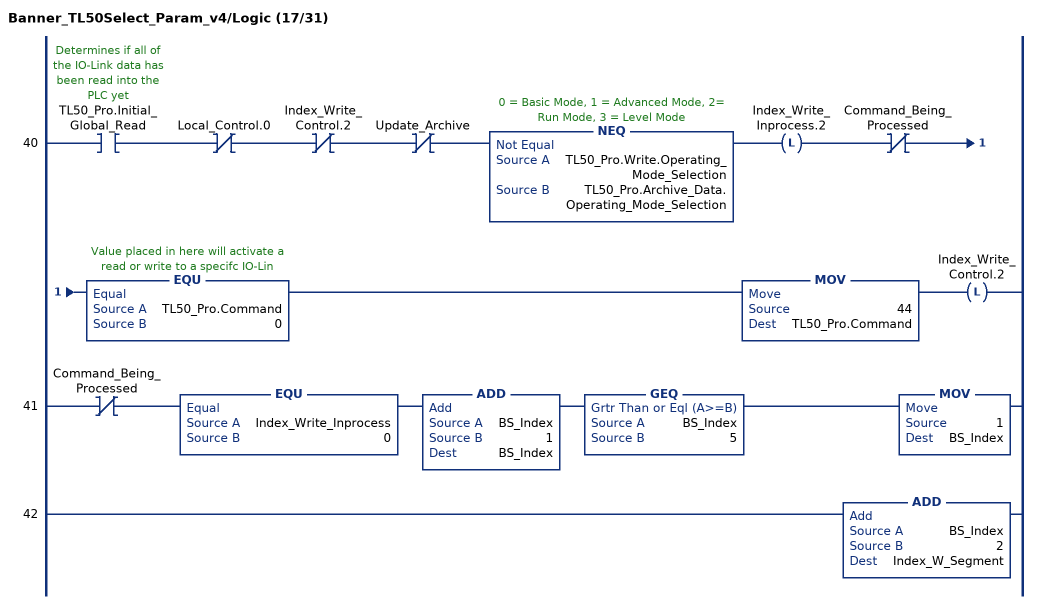
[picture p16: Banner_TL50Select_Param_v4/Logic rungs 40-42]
   40: XIC(TL50_Pro.Initial_Global_Read)XIO(Local_Control.0)XIO(Index_Write_Control.2)XIO(Update_Archive)NEQ(TL50_Pro.Write.Operating_Mode_Selection,TL50_Pro.Archive_Data.Operating_Mode_Selection)OTL(Index_Write_Inprocess.2)XIO(Command_Being_Processed)EQU(TL50_Pro.Command,0)MOV(44,TL50_Pro.Command)OTL(Index_Write_Control.2);
   41: XIO(Command_Being_Processed)EQU(Index_Write_Inprocess,0)ADD(BS_Index,1,BS_Index)GEQ(BS_Index,5)MOV(1,BS_Index);
   42: ADD(BS_Index,2,Index_W_Segment);
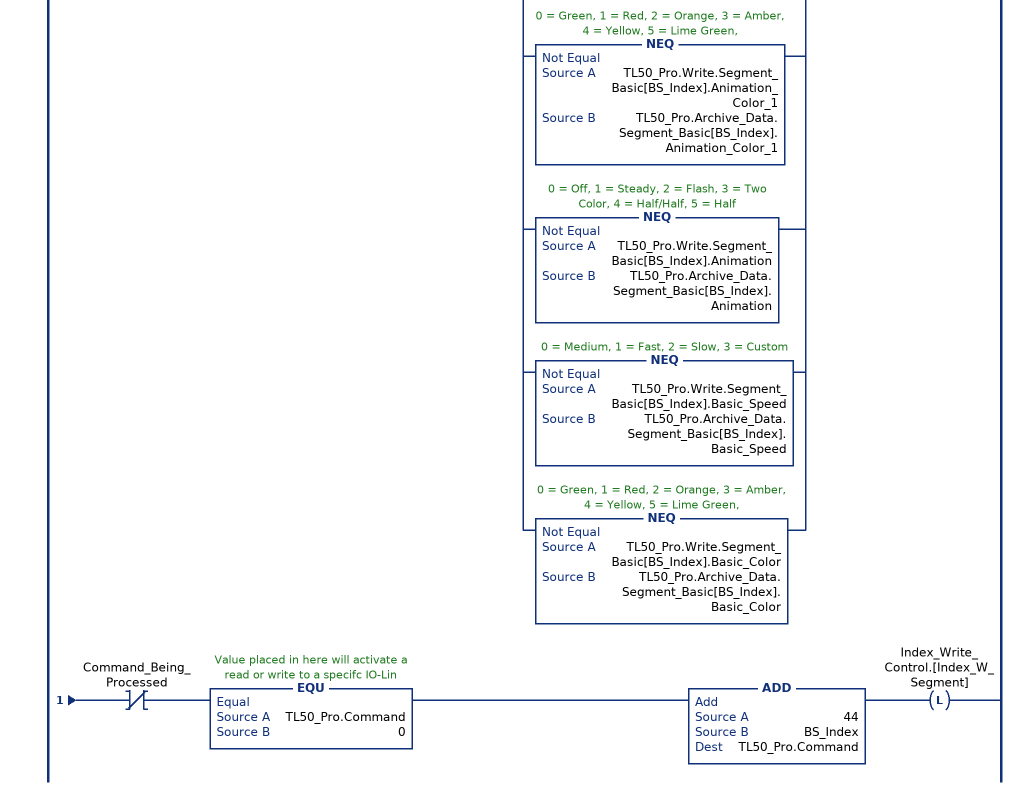
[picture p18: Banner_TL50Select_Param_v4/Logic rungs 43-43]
   43: XIC(TL50_Pro.Initial_Global_Read)XIO(Local_Control.0)XIO(Index_Write_Control.[Index_W_Segment])XIO(Update_Archive)[NEQ(TL50_Pro.Write.Segment_Basic[BS_Index].Animation_Color_2_Intensity,TL50_Pro.Archive_Data.Segment_Basic[BS_Index].Animation_Color_2_Intensity) ,NEQ(TL50_Pro.Write.Segment_Basic[BS_Index].Animation_Color_2,TL50_Pro.Archive_Data.Segment_Basic[BS_Index].Animation_Color_2) ,NEQ(TL50_Pro.Write.Segment_Basic[BS_Index].Animation_Pattern,TL50_Pro.Archive_Data.Segment_Basic[BS_Index].Animation_Pattern) ,NEQ(TL50_Pro.Write.Segment_Basic[BS_Index].Animation_Speed,TL50_Pro.Archive_Data.Segment_Basic[BS_Index].Animation_Speed) ,NEQ(TL50_Pro.Write.Segment_Basic[BS_Index].Animation_Color_1_Intensity,TL50_Pro.Archive_Data.Segment_Basic[BS_Index].Animation_Color_1_Intensity) ,NEQ(TL50_Pro.Write.Segment_Basic[BS_Index].Animation_Color_1,TL50_Pro.Archive_Data.Segment_Basic[BS_Index].Animation_Color_1) ,NEQ(TL50_Pro.Write.Segment_Basic[BS_Index].Animation,TL50_Pro.Archive_Data.Segment_Basic[BS_Index].Animation) ,NEQ(TL50_Pro.Write.Segment_Basic[BS_Index].Basic_Speed,TL50_Pro.Archive_Data.Segment_Basic[BS_Index].Basic_Speed) ,NEQ(TL50_Pro.Write.Segment_Basic[BS_Index].Basic_Color,TL50_Pro.Archive_Data.Segment_Basic[BS_Index].Basic_Color) ]OTL(Index_Write_Inprocess.[Index_W_Segment])XIO(Command_Being_Processed)EQU(TL50_Pro.Command,0)ADD(44,BS_Index,TL50_Pro.Command)OTL(Index_Write_Control.[Index_W_Segment]);
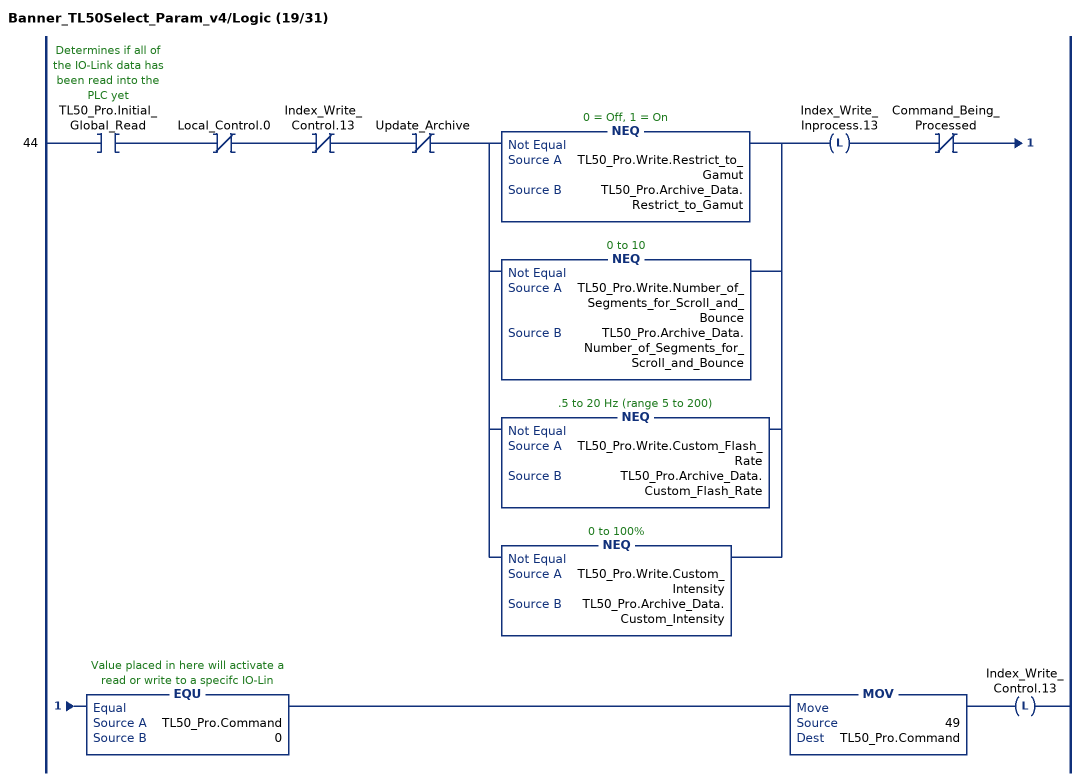
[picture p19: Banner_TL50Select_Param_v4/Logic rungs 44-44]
   44: XIC(TL50_Pro.Initial_Global_Read)XIO(Local_Control.0)XIO(Index_Write_Control.13)XIO(Update_Archive)[NEQ(TL50_Pro.Write.Restrict_to_Gamut,TL50_Pro.Archive_Data.Restrict_to_Gamut) ,NEQ(TL50_Pro.Write.Number_of_Segments_for_Scroll_and_Bounce,TL50_Pro.Archive_Data.Number_of_Segments_for_Scroll_and_Bounce) ,NEQ(TL50_Pro.Write.Custom_Flash_Rate,TL50_Pro.Archive_Data.Custom_Flash_Rate) ,NEQ(TL50_Pro.Write.Custom_Intensity,TL50_Pro.Archive_Data.Custom_Intensity) ]OTL(Index_Write_Inprocess.13)XIO(Command_Being_Processed)EQU(TL50_Pro.Command,0)MOV(49,TL50_Pro.Command)OTL(Index_Write_Control.13);
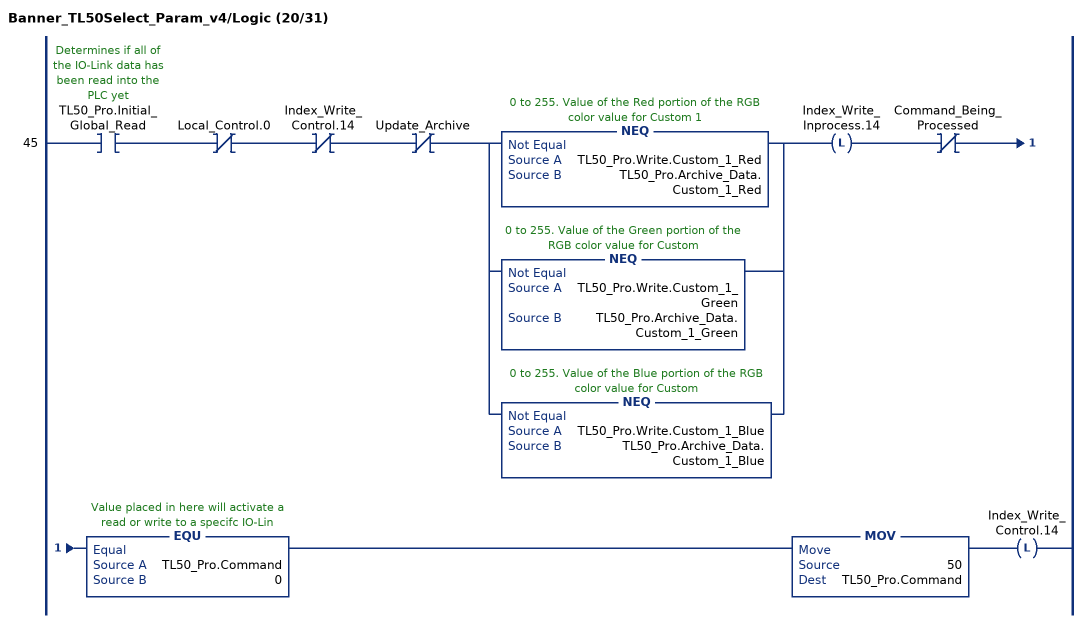
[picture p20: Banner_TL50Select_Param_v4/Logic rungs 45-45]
   45: XIC(TL50_Pro.Initial_Global_Read)XIO(Local_Control.0)XIO(Index_Write_Control.14)XIO(Update_Archive)[NEQ(TL50_Pro.Write.Custom_1_Red,TL50_Pro.Archive_Data.Custom_1_Red) ,NEQ(TL50_Pro.Write.Custom_1_Green,TL50_Pro.Archive_Data.Custom_1_Green) ,NEQ(TL50_Pro.Write.Custom_1_Blue,TL50_Pro.Archive_Data.Custom_1_Blue) ]OTL(Index_Write_Inprocess.14)XIO(Command_Being_Processed)EQU(TL50_Pro.Command,0)MOV(50,TL50_Pro.Command)OTL(Index_Write_Control.14);
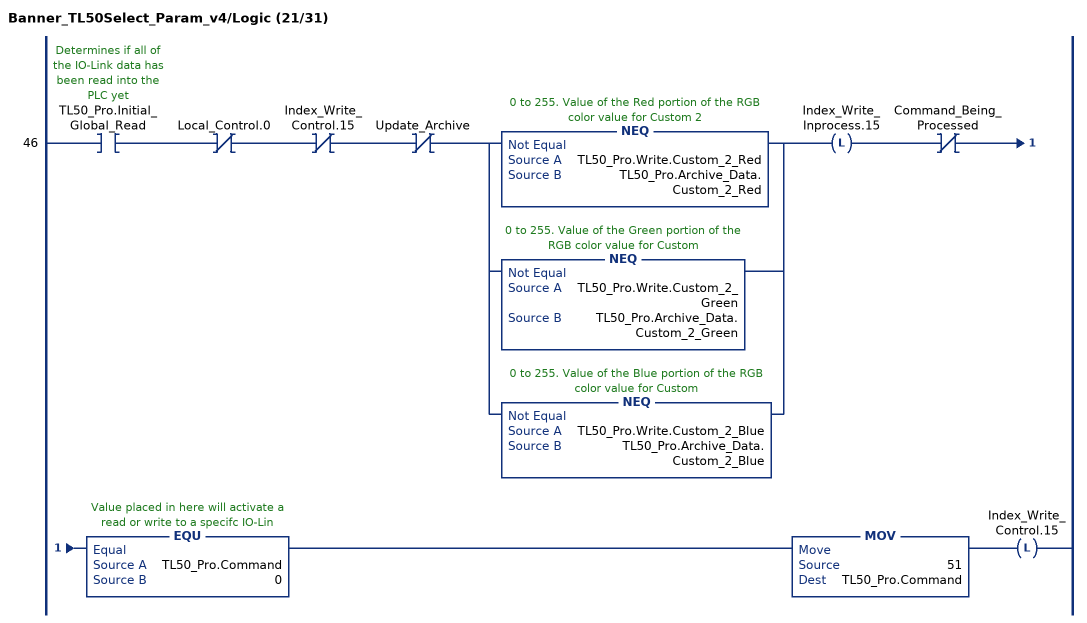
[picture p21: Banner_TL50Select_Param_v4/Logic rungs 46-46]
   46: XIC(TL50_Pro.Initial_Global_Read)XIO(Local_Control.0)XIO(Index_Write_Control.15)XIO(Update_Archive)[NEQ(TL50_Pro.Write.Custom_2_Red,TL50_Pro.Archive_Data.Custom_2_Red) ,NEQ(TL50_Pro.Write.Custom_2_Green,TL50_Pro.Archive_Data.Custom_2_Green) ,NEQ(TL50_Pro.Write.Custom_2_Blue,TL50_Pro.Archive_Data.Custom_2_Blue) ]OTL(Index_Write_Inprocess.15)XIO(Command_Being_Processed)EQU(TL50_Pro.Command,0)MOV(51,TL50_Pro.Command)OTL(Index_Write_Control.15);
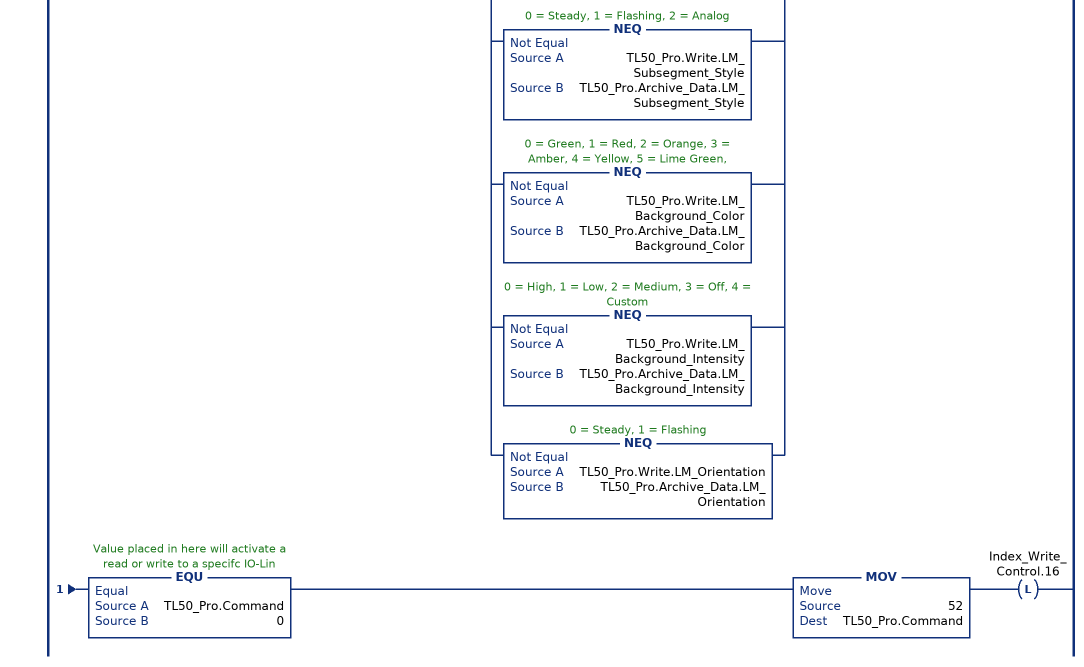
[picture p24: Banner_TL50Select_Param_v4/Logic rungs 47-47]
   47: XIC(TL50_Pro.Initial_Global_Read)XIO(Local_Control.0)XIO(Index_Write_Control.16)XIO(Update_Archive)[NEQ(TL50_Pro.Write.LM_Full_Scale_Value,TL50_Pro.Archive_Data.LM_Full_Scale_Value) ,NEQ(TL50_Pro.Write.LM_Base_Color,TL50_Pro.Archive_Data.LM_Base_Color) ,NEQ(TL50_Pro.Write.LM_Base_Intensity,TL50_Pro.Archive_Data.LM_Base_Intensity) ,NEQ(TL50_Pro.Write.LM_Base_State,TL50_Pro.Archive_Data.LM_Base_State) ,NEQ(TL50_Pro.Write.LM_Threshold_Type,TL50_Pro.Archive_Data.LM_Threshold_Type) ,NEQ(TL50_Pro.Write.LM_Low_Threshold_Value,TL50_Pro.Archive_Data.LM_Low_Threshold_Value) ,NEQ(TL50_Pro.Write.LM_Low_Threshold_Color,TL50_Pro.Archive_Data.LM_Low_Threshold_Color) ,NEQ(TL50_Pro.Write.LM_Low_Threshold_Intensity,TL50_Pro.Archive_Data.LM_Low_Threshold_Intensity) ,NEQ(TL50_Pro.Write.LM_Low_Threshold_State,TL50_Pro.Archive_Data.LM_Low_Threshold_State) ,NEQ(TL50_Pro.Write.LM_High_Threshold_Value,TL50_Pro.Archive_Data.LM_High_Threshold_Value) ,NEQ(TL50_Pro.Write.LM_High_Threshold_Color,TL50_Pro.Archive_Data.LM_High_Threshold_Color) ,NEQ(TL50_Pro.Write.LM_High_Threshold_Intensity,TL50_Pro.Archive_Data.LM_High_Threshold_Intensity) ,NEQ(TL50_Pro.Write.LM_High_Threshold_State,TL50_Pro.Archive_Data.LM_High_Threshold_State) ,NEQ(TL50_Pro.Write.LM_Flash_Rate,TL50_Pro.Archive_Data.LM_Flash_Rate) ,NEQ(TL50_Pro.Write.LM_Dominance,TL50_Pro.Archive_Data.LM_Dominance) ,NEQ(TL50_Pro.Write.LM_Subsegment_Style,TL50_Pro.Archive_Data.LM_Subsegment_Style) ,NEQ(TL50_Pro.Write.LM_Background_Color,TL50_Pro.Archive_Data.LM_Background_Color) ,NEQ(TL50_Pro.Write.LM_Background_Intensity,TL50_Pro.Archive_Data.LM_Background_Intensity) ,NEQ(TL50_Pro.Write.LM_Orientation,TL50_Pro.Archive_Data.LM_Orientation) ]OTL(Index_Write_Inprocess.16)XIO(Command_Being_Processed)EQU(TL50_Pro.Command,0)MOV(52,TL50_Pro.Command)OTL(Index_Write_Control.16);
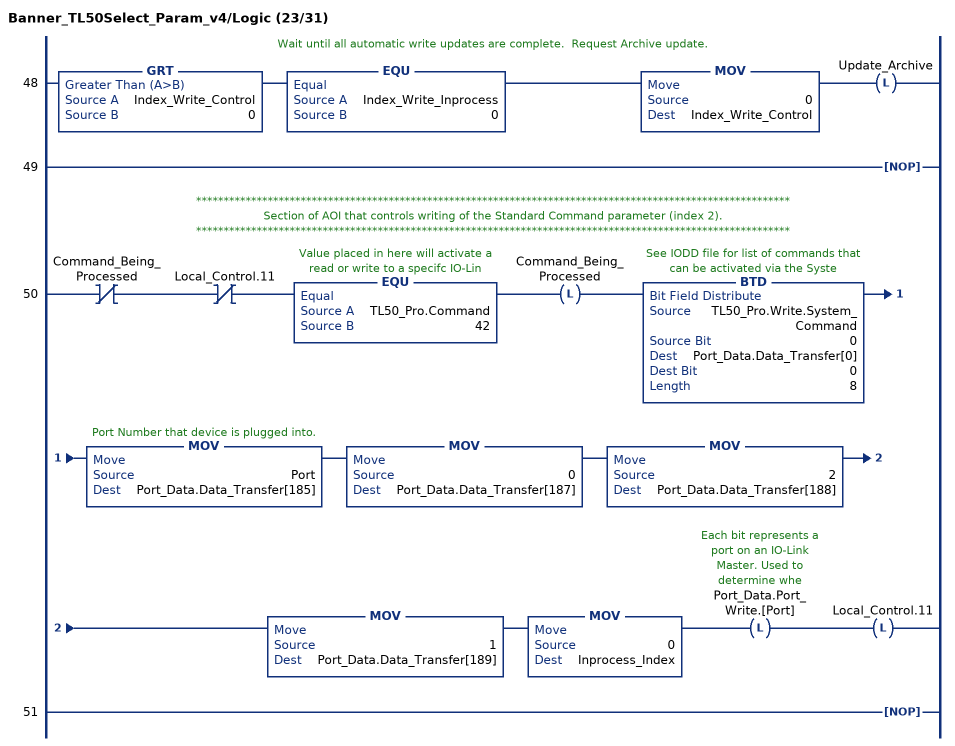
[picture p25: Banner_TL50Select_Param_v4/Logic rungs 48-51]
   // Wait until all automatic write updates are complete.  Request Archive update.
   48: GRT(Index_Write_Control,0)EQU(Index_Write_Inprocess,0)MOV(0,Index_Write_Control)OTL(Update_Archive);
   49: NOP();
   // ************************************************************************************************************
   // Section of AOI that controls writing of the Standard Command parameter (index 2).
   // ************************************************************************************************************
   50: XIO(Command_Being_Processed)XIO(Local_Control.11)EQU(TL50_Pro.Command,42)OTL(Command_Being_Processed)BTD(TL50_Pro.Write.System_Command,0,Port_Data.Data_Transfer[0],0,8)MOV(Port,Port_Data.Data_Transfer[185])MOV(0,Port_Data.Data_Transfer[187])MOV(2,Port_Data.Data_Transfer[188])MOV(1,Port_Data.Data_Transfer[189])MOV(0,Inprocess_Index)OTL(Port_Data.Port_Write.[Port])OTL(Local_Control.11);
   51: NOP();
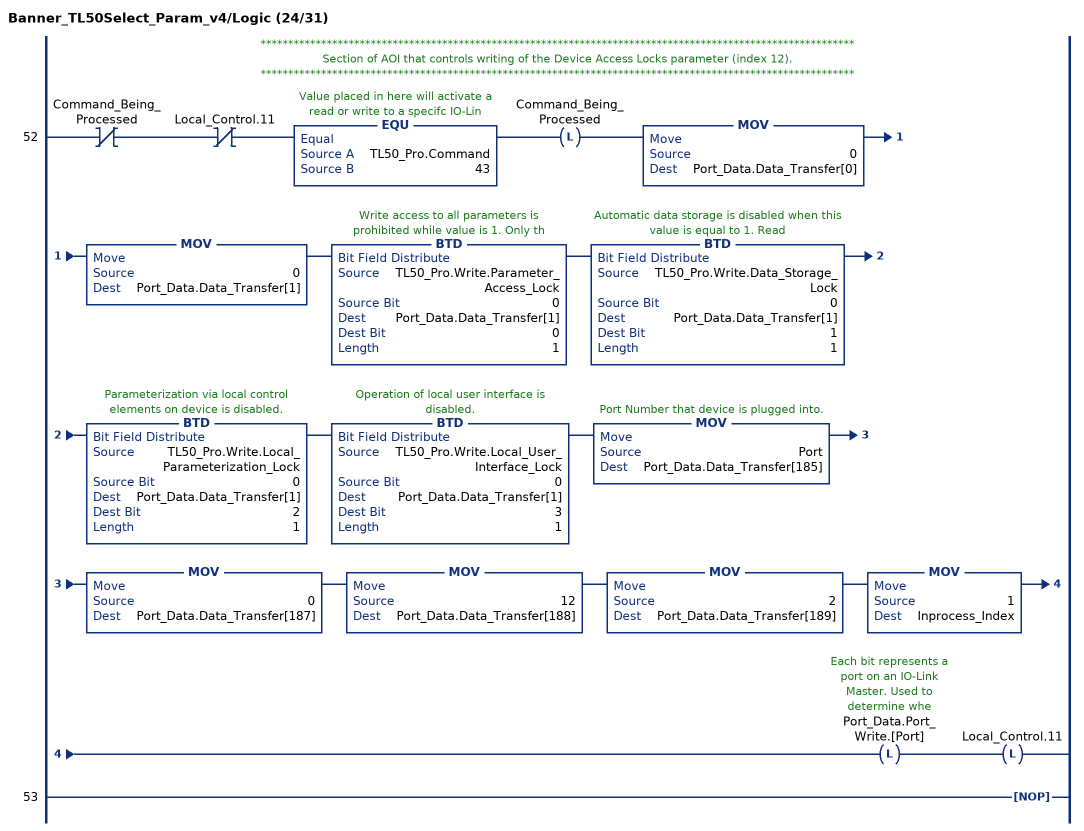
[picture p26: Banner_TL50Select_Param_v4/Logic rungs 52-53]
   // ************************************************************************************************************
   // Section of AOI that controls writing of the Device Access Locks parameter (index 12).
   // ************************************************************************************************************
   52: XIO(Command_Being_Processed)XIO(Local_Control.11)EQU(TL50_Pro.Command,43)OTL(Command_Being_Processed)MOV(0,Port_Data.Data_Transfer[0])MOV(0,Port_Data.Data_Transfer[1])BTD(TL50_Pro.Write.Parameter_Access_Lock,0,Port_Data.Data_Transfer[1],0,1)BTD(TL50_Pro.Write.Data_Storage_Lock,0,Port_Data.Data_Transfer[1],1,1)BTD(TL50_Pro.Write.Local_Parameterization_Lock,0,Port_Data.Data_Transfer[1],2,1)BTD(TL50_Pro.Write.Local_User_Interface_Lock,0,Port_Data.Data_Transfer[1],3,1)MOV(Port,Port_Data.Data_Transfer[185])MOV(0,Port_Data.Data_Transfer[187])MOV(12,Port_Data.Data_Transfer[188])MOV(2,Port_Data.Data_Transfer[189])MOV(1,Inprocess_Index)OTL(Port_Data.Port_Write.[Port])OTL(Local_Control.11);
   53: NOP();
